(* Logix 5000 AddOnInstructionDefinition export AMCI_SD4840E2_Axis_Follower_Circular; software revision 20.03 *)

ADD_ON_INSTRUCTION AMCI_SD4840E2_Axis_Follower_Circular   (* revision 1.0, vendor AMCI, ExecuteEnableInFalse *)
VAR_INPUT
   Axis_Status_Bits : INT; {required}
   Follower_Type_Motor_or_Encoder : BOOL; {required}
   Follower_Position : REAL; {required}
   Follower_Velocity : REAL; {required}
   Acceleration : INT; {required}
   Deceleration : INT; {required}
   Proportional_Coefficient : INT; {required}
   Conversion_Constant : REAL; {required}
   Position_Unwind : INT; {required}
END_VAR
VAR_IN_OUT
   AMCI_SD4840E2_output_data : _000A:SD4840E2_4342D302:O:0; {required}
END_VAR
VAR_OUTPUT
   EN : BOOL; {visible}
   Axis_Follower_occurring : BOOL; {visible}
   ER : BOOL; {visible}
END_VAR
VAR
   command_data_block : INT[10];
        [0]   // Command Bits MSW
        [1]   // Command Bits LSW
        [2]   // Upper Target Position
        [3]   // Lower Target Position
        [4]   // Upper Programmed Speed
        [5]   // Lower Programmed Speed
   axis_follower_position : DINT;
   axis_follower_velocity : DINT;
END_VAR

ROUTINE EnableInFalse   (* ladder *)
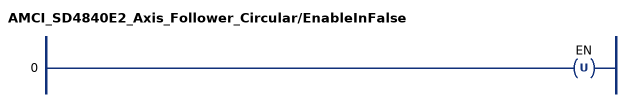
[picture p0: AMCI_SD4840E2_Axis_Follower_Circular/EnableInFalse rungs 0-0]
   0: OTU(EN);
END_ROUTINE

ROUTINE Logic   (* ladder *)
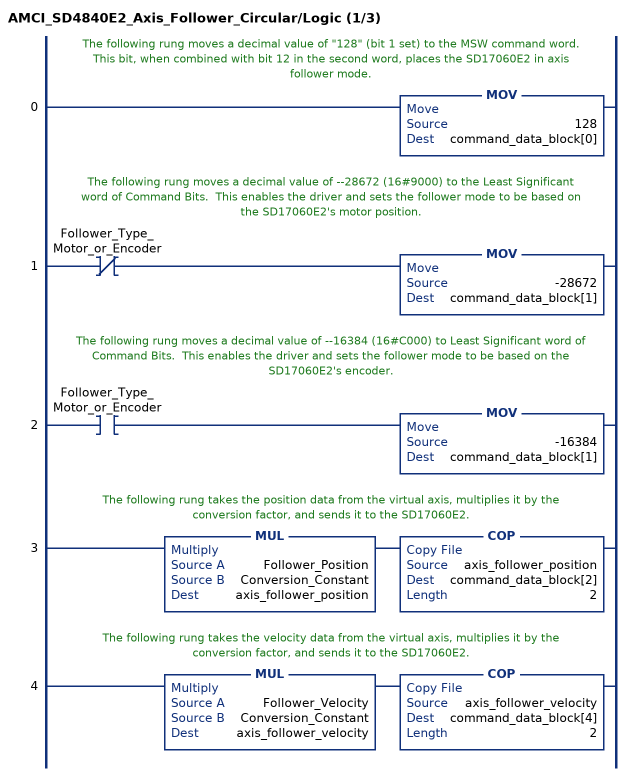
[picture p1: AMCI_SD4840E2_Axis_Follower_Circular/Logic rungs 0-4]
   // The following rung moves a decimal value of "128" (bit 1 set) to the MSW command word.  This bit, when combined with bit 12 in the second word, places the SD17060E2 in axis follower mode.
   0: MOV(128,command_data_block[0]);
   // The following rung moves a decimal value of --28672 (16#9000) to the Least Significant word of Command Bits.  This enables the driver and sets the follower mode to be based on the SD17060E2's motor position.
   1: XIO(Follower_Type_Motor_or_Encoder)MOV(-28672,command_data_block[1]);
   // The following rung moves a decimal value of --16384 (16#C000) to Least Significant word of Command Bits.  This enables the driver and sets the follower mode to be based on the SD17060E2's encoder.
   2: XIC(Follower_Type_Motor_or_Encoder)MOV(-16384,command_data_block[1]);
   // The following rung takes the position data from the virtual axis, multiplies it by the conversion factor, and sends it to the SD17060E2.
   3: MUL(Follower_Position,Conversion_Constant,axis_follower_position)COP(axis_follower_position,command_data_block[2],2);
   // The following rung takes the velocity data from the virtual axis, multiplies it by the conversion factor, and sends it to the SD17060E2.
   4: MUL(Follower_Velocity,Conversion_Constant,axis_follower_velocity)COP(axis_follower_velocity,command_data_block[4],2);
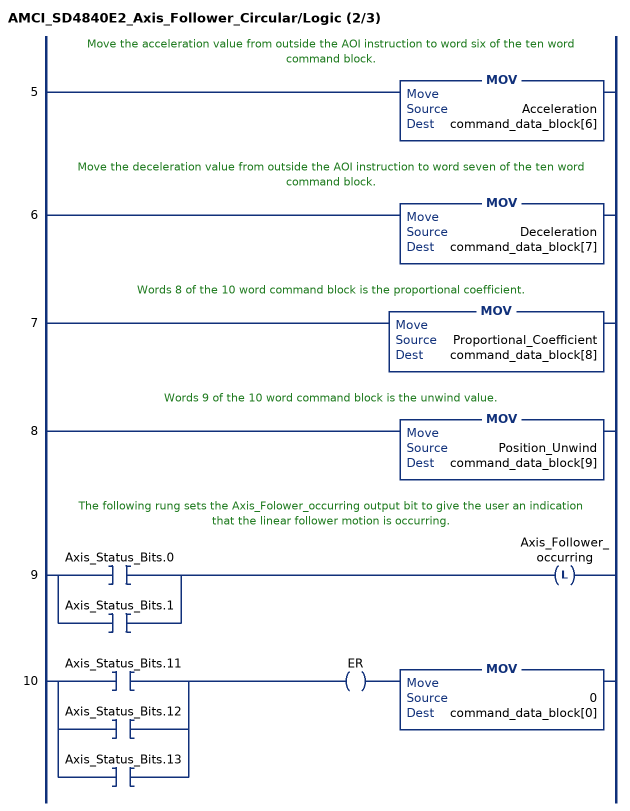
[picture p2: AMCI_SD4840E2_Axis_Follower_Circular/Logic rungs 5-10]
   // Move the acceleration value from outside the AOI instruction to word six of the ten word command block.
   5: MOV(Acceleration,command_data_block[6]);
   // Move the deceleration value from outside the AOI instruction to word seven of the ten word command block.
   6: MOV(Deceleration,command_data_block[7]);
   // Words 8 of the 10 word command block is the proportional coefficient.
   7: MOV(Proportional_Coefficient,command_data_block[8]);
   // Words 9 of the 10 word command block is the unwind value.
   8: MOV(Position_Unwind,command_data_block[9]);
   // The following rung sets the Axis_Folower_occurring output bit to give the user an indication that the linear follower motion is occurring.
   9: [XIC(Axis_Status_Bits.0) ,XIC(Axis_Status_Bits.1) ]OTL(Axis_Follower_occurring);
   10: [XIC(Axis_Status_Bits.11) ,XIC(Axis_Status_Bits.12) ,XIC(Axis_Status_Bits.13) ]OTE(ER)MOV(0,command_data_block[0]);
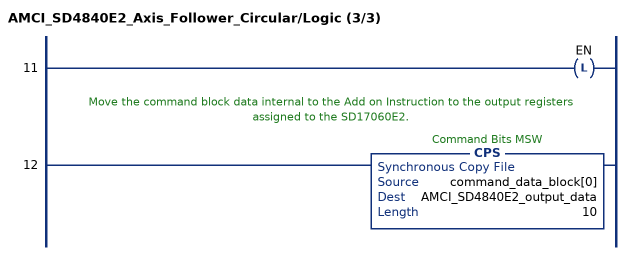
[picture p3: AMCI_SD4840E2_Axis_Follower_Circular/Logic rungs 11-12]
   11: OTL(EN);
   // Move the command block data internal to the Add on Instruction to the output registers assigned to the SD17060E2.
   12: CPS(command_data_block[0],AMCI_SD4840E2_output_data,10);
END_ROUTINE
END_ADD_ON_INSTRUCTION
